FUNCTION "FC RIC. TEMP INGRESSO WD" : VOID
TITLE =FC RICHIAMO PER GESTIONE TEMPERATURA WORK DESK
{ S7_language := '16(1) Italiano (Italia)  24.10.2008  14:50:58' }
AUTHOR : Hofmann
FAMILY : Av
NAME : Av_RdSca
VERSION : 1.3


VAR_INPUT
  AVal : WORD ;	//Valore effettivo analogico per gli input dalla periferia (PEW/EW)
  HI_LIM : REAL ;	//Limite superiore fisico (e.g. 600°C/100%)
  LO_LIM : REAL ;	//Limite inferiore fisico (e.g. 0°C/0%)
  CBIP : BOOL ;	//Controllo bit di input bipolare (0=unipolare/1=bipolare)
  Repl : REAL ;	//Valore di sostituzione del valore effettivo in caso di allarme
END_VAR
VAR_OUTPUT
  AVa : REAL ;	//Output standard del valore analogico (e.g. In °C/%)
  FBW : BOOL ;	//Valore effettivo dell'Allarme di bit (circuito ele. interrotto, 0=All./ 1=OK)
END_VAR
VAR_TEMP
  H1_AVPer : INT ;	//Valore effettivo dalla periferia
  H1_AVTemp : REAL ;	//Valore effettivo temporaneo
  H1_RET_VAL : WORD ;	//allarme di informazione dell'evento
END_VAR
BEGIN
NETWORK
TITLE =nuova sonda temperaura
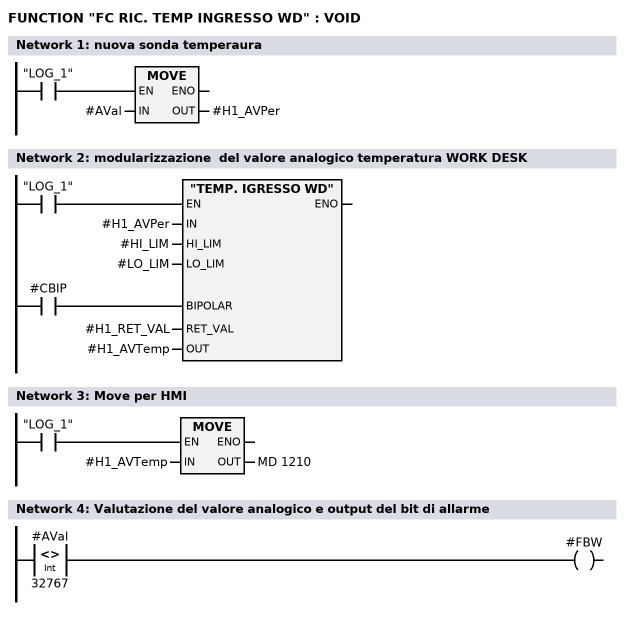
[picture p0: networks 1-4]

      U     "LOG_1";
      SPBNB _001;
      L     #AVal;
      T     #H1_AVPer;
_001: NOP   0;
NETWORK
TITLE =modularizzazione  del valore analogico temperatura WORK DESK

      U     #CBIP;
      =     L      8.0;
      BLD   103;
      U     "LOG_1";
      SPBNB _002;
      CALL "TEMP. IGRESSO WD" (
           IN                       := #H1_AVPer,
           HI_LIM                   := #HI_LIM,
           LO_LIM                   := #LO_LIM,
           BIPOLAR                  := L      8.0,
           RET_VAL                  := #H1_RET_VAL,
           OUT                      := #H1_AVTemp);
_002: NOP   0;
NETWORK
TITLE =Move per HMI

      U     "LOG_1";
      SPBNB _003;
      L     #H1_AVTemp;
      T     MD  1210;
_003: NOP   0;
NETWORK
TITLE =Valutazione del valore analogico e output del bit di allarme

      L     #AVal;
      L     32767;
      <>I   ;
      =     #FBW;
NETWORK
TITLE =Output del valore analogico

      UN    #FBW;
      SPB   M001;
// ;
      L     #H1_AVTemp;
      T     #AVa;
      SPA   M002;
// ;
M001: L     #Repl;
      T     #AVa;
M002: NOP   0;
NETWORK
TITLE =impostazione abilitare ENO

      SET   ;
      SAVE  ;
END_FUNCTION

